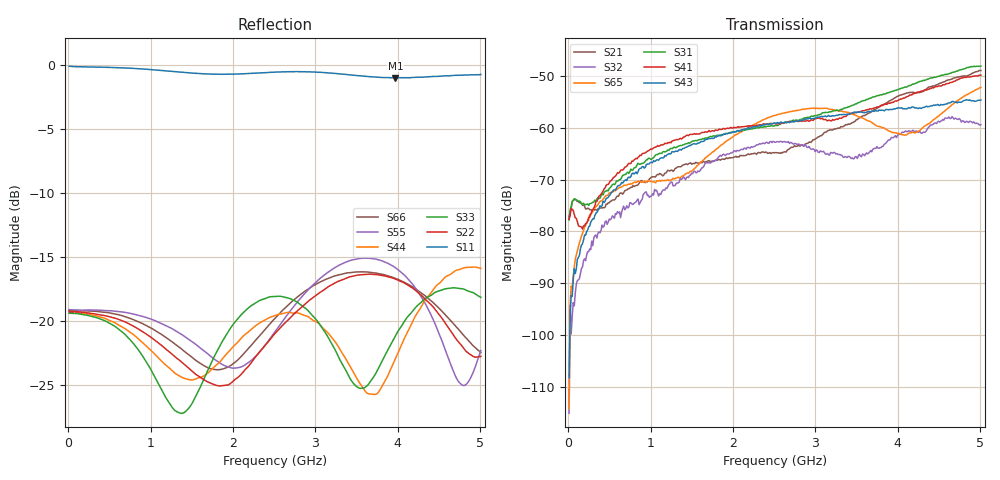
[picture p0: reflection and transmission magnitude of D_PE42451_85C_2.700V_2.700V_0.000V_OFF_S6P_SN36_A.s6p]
! Device ID: PE42451
! Serial: 36
! Insertion: A
! Temp: 85C
! VDD: 2.700
! Control_Hi: 100.000
! Control_Lo: 0.000
! Logic State: OFF
! Port 1: RFC
! Port 2: RF1
! Port 3: RF2
! Port 4: RF3
! Port 5: RF4
! Port 6: RF5
! V1 = 0.00
! V2 = 2.70
! V3 = 2.70
! V4 = 0.00
! IDD: 1.130170e-05
#  Hz  S  RI  R  50
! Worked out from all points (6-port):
!   401 points, 10 MHz to 5.01 GHz, reference 50 ohm
!   strongest paths, dB at 10 MHz, 1.26 GHz, 2.51 GHz, 3.76 GHz, 5.01 GHz:
!     S43: -108.2, -64.6, -59.1, -56.8, -54.6
!     S41: -77.7, -62.5, -59.1, -56.0, -49.8
!     S31: -77.8, -64.0, -59.5, -53.8, -48.1
!     S65: -114.2, -70.0, -57.6, -59.7, -52.2
!     S32: -115.1, -70.5, -62.8, -63.9, -59.4
!     S21: -77.2, -68.2, -64.8, -56.1, -48.9
!   lowest |S11| = -1.0 dB at 3.973 GHz (marker M1), VSWR 16.91, Z = 3.19 - j14 ohm
!   |S11| at or under -10 dB: nowhere
